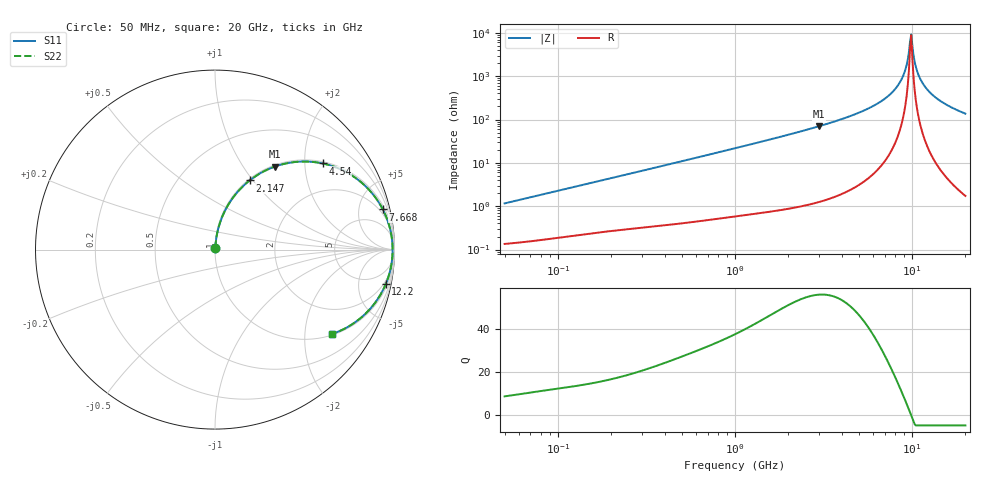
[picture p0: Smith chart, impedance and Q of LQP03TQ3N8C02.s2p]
!Murata Part Number: LQP03TQ3N8C02
!These Parameters are Measured in Series Mode Connection
!  o--[Z]--o
!Port1  Port2
!  o-------o
!Freq. Start=50[MHz] Stop=20[GHz], 401[Steps]
# Hz S RI R 50
!Freq.(Hz) S11(Real) S11(Imag) S21(Real) S21(Imag) S12(Real) S12(Imag) S22(Real) S22(Imag)
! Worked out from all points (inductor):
!   401 points, 50 MHz to 20 GHz, reference 50 ohm
!   read as one part in series: L = 3.65 nH near 51.52 MHz
!   highest Q = 56 at 2.985 GHz (marker M1), where L = 3.74 nH
!   self-resonance near 9.745 GHz
!   S11 on the Smith chart (normalised r, x): 50 MHz: 1.00, +0.02; 2.147 GHz: 1.02, +0.96; 4.54 GHz: 1.05, +2.45; 7.668 GHz: 1.39, +8.25; 12.2 GHz: 1.47, -9.76; 20 GHz: 1.03, -2.73
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5e7  0.00148 0.0115  0.9985 -0.0115  0.9985 -0.0115  0.00148 0.0115
1.364002e8  0.00314 0.0305  0.9969 -0.0305  0.9969 -0.0305  0.00314 0.0305
3.721004e8  0.01 0.0803  0.99 -0.0803  0.99 -0.0803  0.01 0.0803
1e9  0.0501 0.2053  0.9499 -0.2053  0.9499 -0.2053  0.0501 0.2053
2.146657e9  0.1927 0.385  0.8073 -0.385  0.8073 -0.385  0.1927 0.385
2.728004e9  0.2878 0.4438  0.7122 -0.4438  0.7122 -0.4438  0.2878 0.4438
2.98453e9  0.3322 0.4621  0.6678 -0.4621  0.6678 -0.4621  0.3322 0.4621
4.539627e9  0.5991 0.4802  0.4009 -0.4802  0.4009 -0.4802  0.5991 0.4802
6.034176e9  0.8021 0.3852  0.1979 -0.3852  0.1979 -0.3852  0.8021 0.3852
7.442007e9  0.9221 0.2474  0.0779 -0.2474  0.0779 -0.2474  0.9221 0.2474
7.668323e9  0.9352 0.2237  0.0648 -0.2237  0.0648 -0.2237  0.9352 0.2237
8.389408e9  0.9665 0.1477  0.0335 -0.1477  0.0335 -0.1477  0.9665 0.1477
8.907419e9  0.9803 0.094  0.0197 -0.094  0.0197 -0.094  0.9803 0.094
9.316812e9  0.9867 0.0527  0.0133 -0.0527  0.0133 -0.0527  0.9867 0.0527
9.600142e9  0.989 0.0249  0.011 -0.0249  0.011 -0.0249  0.989 0.0249
9.892087e9  0.9897 -0.00307  0.0103 0.00307  0.0103 0.00307  0.9897 -0.00307
1.004137e10  0.9894 -0.017  0.0106 0.017  0.0106 0.017  0.9894 -0.017
1.050288e10  0.9863 -0.0588  0.0137 0.0588  0.0137 0.0588  0.9863 -0.0588
1.082228e10  0.9823 -0.0864  0.0177 0.0864  0.0177 0.0864  0.9823 -0.0864
1.220001e10  0.9512 -0.1926  0.0488 0.1926  0.0488 0.1926  0.9512 -0.1926
1.504638e10  0.8475 -0.3482  0.1525 0.3482  0.1525 0.3482  0.8475 -0.3482
2e10  0.6496 -0.4708  0.3504 0.4708  0.3504 0.4708  0.6496 -0.4708
